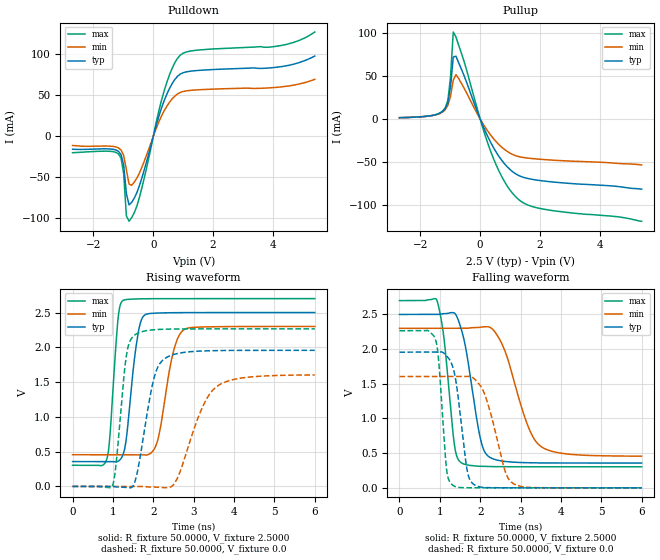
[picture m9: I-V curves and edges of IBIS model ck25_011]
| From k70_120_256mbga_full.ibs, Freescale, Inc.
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|   Model ck25_011
[Model]  ck25_011
Model_type Output
Polarity   Non-Inverting
Enable   Active-High
Vmeas =  1.2500V
Cref =   5.0000pF
Rref =   50.0000
C_comp   2.8000pF   2.5000pF   3.3000pF
[Temperature Range]   25.0000   0.1250k   -40.0000
[Voltage Range]   2.5000V   2.3000V   2.7000V
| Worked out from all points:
|   slope of the pulldown table from 0 to 0.375 V, typ, clamps not added: 8.44 ohm
|   slope of the pullup table from 0 to 0.375 V, typ, clamps not added: 13 ohm
|   rising waveform, R_fixture 50.0000, V_fixture 2.5000: 20-80 % time 236ps typ, 325ps min, 165ps max; typ from 0.357 V to 2.5 V
|   rising waveform, R_fixture 50.0000, V_fixture 0.0: 20-80 % time 356ps typ, 616ps min, 215ps max; typ from 0 V to 1.96 V
|   falling waveform, R_fixture 50.0000, V_fixture 2.5000: 20-80 % time 354ps typ, 590ps min, 239ps max; typ from 2.5 V to 0.357 V
|   falling waveform, R_fixture 50.0000, V_fixture 0.0: 20-80 % time 250ps typ, 427ps min, 163ps max; typ from 1.96 V to 0 V
[Pulldown]
|Voltage   I(typ)   I(min)   I(max)
-2.7V     -15.77mA   -11.2mA    -19.98mA
-1.17V    -18.13mA   -14.01mA   -21.28mA
-1.08V    -22.19mA   -16.64mA   -26.33mA
-990mV    -35.18mA   -23.44mA   -45.79mA
-900mV    -69.88mA   -40.78mA   -97.1mA
-810mV    -83.67mA   -58.35mA   -103.6mA
-450mV    -58.65mA   -43.63mA   -72.59mA
360mV     43.1mA     30.89mA    55.11mA
630mV     64.27mA    45.66mA    82.94mA
900mV     75.87mA    53.52mA    98.99mA
4.23V     84.8mA     60.1mA     110.5mA
5.4V      97.9mA     69.5mA     127.2mA
[Pullup]
|Voltage   I(typ)   I(min)   I(max)
-2.7V     1.5mA      1.5mA      1.5mA
-1.53V    4.63mA     4.47mA     4.69mA
-1.17V    12.09mA    10.79mA    12.86mA
-1.08V    19.13mA    15.88mA    21.56mA
-990mV    37.69mA    26.64mA    49.85mA
-900mV    72.26mA    45.45mA    101.4mA
-720mV    65.74mA    47.23mA    86.18mA
360mV     -27.88mA   -19.21mA   -38.56mA
720mV     -48.14mA   -32.87mA   -67.14mA
1.17V     -63.58mA   -42.61mA   -90.14mA
1.98V     -71.69mA   -46.92mA   -104.2mA
5.4V      -81.9mA    -53.62mA   -119.3mA
[Ramp]
| variable   typ   min   max
dV/dt_r  1.1739/0.3562n   0.9617/0.6155n   1.3590/0.2154n
dV/dt_f  1.2856/0.3544n   1.1060/0.5899n   1.4377/0.2386n
R_load = 50.0000
[Rising Waveform]
R_fixture= 50.0000
V_fixture= 2.5000
V_fixture_min= 2.3000
V_fixture_max= 2.7000
|time   V(typ)   V(min)   V(max)
0s        357.4mV    455.5mV    303.8mV
846.2ps   357.4mV    455.5mV    387.7mV
1.128ns   361.9mV    455.5mV    2.416V
1.244ns   447.6mV    455.5mV    2.671V
1.606ns   2.137V     455.5mV    2.696V
1.784ns   2.462V     452.2mV    2.698V
2.092ns   2.492V     629.7mV    2.699V
2.483ns   2.497V     1.903V     2.7V
2.744ns   2.499V     2.246V     2.7V
6ns       2.5V       2.3V       2.7V
[Rising Waveform]
R_fixture= 50.0000
V_fixture= 0.0
|time   V(typ)   V(min)   V(max)
0s        2.976nV    288.7nV    923.6pV
991.2ps   412.4uV    280.8nV    10.92mV
1.331ns   -17.08mV   1.924uV    1.873V
1.558ns   93.78mV    -59.44uV   2.184V
1.998ns   1.51V      -8.428mV   2.251V
2.298ns   1.843V     -18.9mV    2.26V
2.584ns   1.909V     102.5mV    2.263V
3.165ns   1.946V     1.068V     2.265V
3.555ns   1.952V     1.428V     2.265V
6ns       1.956V     1.603V     2.265V
[Falling Waveform]
R_fixture= 50.0000
V_fixture= 2.5000
V_fixture_min= 2.3000
V_fixture_max= 2.7000
|time   V(typ)   V(min)   V(max)
0s        2.5V       2.3V       2.7V
933.1ps   2.5V       2.3V       2.696V
1.104ns   2.512V     2.3V       2.157V
1.371ns   2.515V     2.3V       583.4mV
1.543ns   2.265V     2.3V       357.1mV
1.986ns   763.7mV    2.315V     311.2mV
2.207ns   452.9mV    2.321V     306.9mV
2.56ns    384.8mV    2.049V     304.6mV
3.484ns   359.5mV    606.2mV    303.9mV
6ns       357.4mV    456.6mV    303.8mV
[Falling Waveform]
R_fixture= 50.0000
V_fixture= 0.0
|time   V(typ)   V(min)   V(max)
0s        1.956V     1.605V     2.265V
897ps     1.956V     1.605V     2.132V
976.4ps   1.957V     1.605V     1.802V
1.166ns   1.902V     1.605V     275.4mV
1.337ns   1.712V     1.605V     30.98mV
1.673ns   267.8mV    1.605V     1.717mV
1.857ns   43.64mV    1.571V     855.8uV
2.115ns   4.481mV    1.343V     317.2uV
2.822ns   458.9uV    61.18mV    21uV
6ns       182nV      15.56uV    -15.67nV
